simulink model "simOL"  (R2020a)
settings: Solver=ode15s  StartTime=0.0  StopTime=tsim  MaxStep=1  RelTol=1e-3
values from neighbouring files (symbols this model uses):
  dnom = [T0nom; TDnom; qDnom; d4nom]    [runOL.m]
  p = [V1;V2;rho;cp;A1;A2;tau01; tau02;transf;MV]    [runOL.m]    (also in Main.m = [N, Fc0, rhoc, rhoh,U,A,cpc,cph]; Main_OL.m = [N, Fc0, rhoc, rhoh,U,A,cpc,cph]; runTestCalcBlk.m = [N, Fc0, rhoc, rhoh,U,A,cpc,cph]; NonlinearMap.m = [U;A;Fc(i);Fh;cpc;cph;Tcin;Thin])
  Tnom = [T1nom;T2nom]    [runOL.m]
  tstep_u = 1000    [runOL.m]
  unom = Qnom    (= 1672)    [runOL.m]
  ustep = unom*1.1    (= 1839.2)    [runOL.m]
undefined symbols (not defined in the file or in its folder): CalcBlock_v, Tank

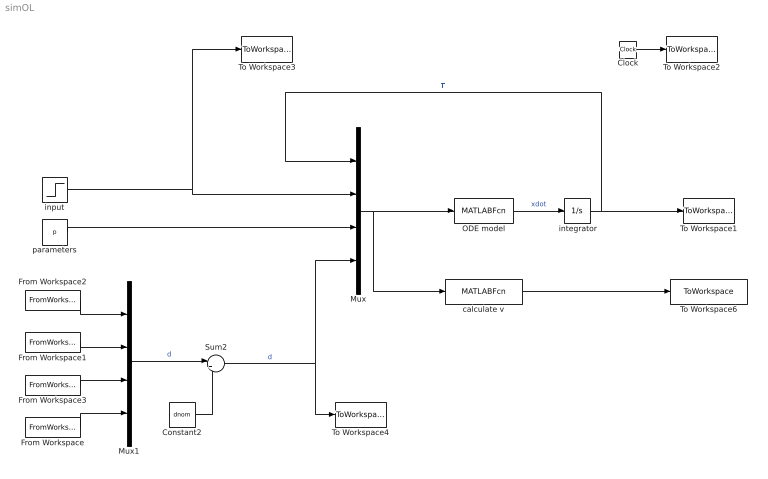
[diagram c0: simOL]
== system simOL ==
  " integrator" : Integrator  InitialCondition=Tnom
  Clock : Clock
  Constant2 : Constant  Value=dnom
  From Workspace : FromWorkspace  VariableName=dist{4}  OutputAfterFinalValue=Setting to zero
  From Workspace1 : FromWorkspace  VariableName=dist{2}  OutputAfterFinalValue=Setting to zero
  From Workspace2 : FromWorkspace  VariableName=dist{1}  OutputAfterFinalValue=Setting to zero
  From Workspace3 : FromWorkspace  VariableName=dist{3}  OutputAfterFinalValue=Setting to zero
  Mux : Mux
  Mux1 : Mux
  ODE model : MATLABFcn  MATLABFcn=Tank(u(1:2), u(3),u(4:13),u(14:17))  OutputDimensions=2
  Sum2 : Sum  Inputs=|++
  To Workspace1 : ToWorkspace  VariableName=T  SampleTime=-1
  To Workspace2 : ToWorkspace  VariableName=time  SampleTime=-1
  To Workspace3 : ToWorkspace  VariableName=u  SampleTime=-1
  To Workspace4 : ToWorkspace  VariableName=d  SampleTime=-1
  To Workspace6 : ToWorkspace  VariableName=vc  SampleTime=-1
  calculate v : MATLABFcn  MATLABFcn=CalcBlock_v(u(1:2), u(3),u(4:13),u(14:17))  OutputDimensions=1
  input : Step  Time=tstep_u  Before=unom  After=ustep  SampleTime=0
  parameters : Constant  Value=p
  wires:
  " integrator"/1 -> Mux/1, To Workspace1/1  "T"
  Clock/1 -> To Workspace2/1
  ODE model/1 -> " integrator"/1  "xdot"
  Sum2/1 -> Mux/4, To Workspace4/1  "d"
  parameters/1 -> Mux/3
  input/1 -> To Workspace3/1, Mux/2
  From Workspace1/1 -> Mux1/2
  From Workspace/1 -> Mux1/4
  From Workspace3/1 -> Mux1/3
  Constant2/1 -> Sum2/2
  Mux1/1 -> Sum2/1  "d"
  From Workspace2/1 -> Mux1/1
  calculate v/1 -> To Workspace6/1
  Mux/1 -> calculate v/1, ODE model/1
